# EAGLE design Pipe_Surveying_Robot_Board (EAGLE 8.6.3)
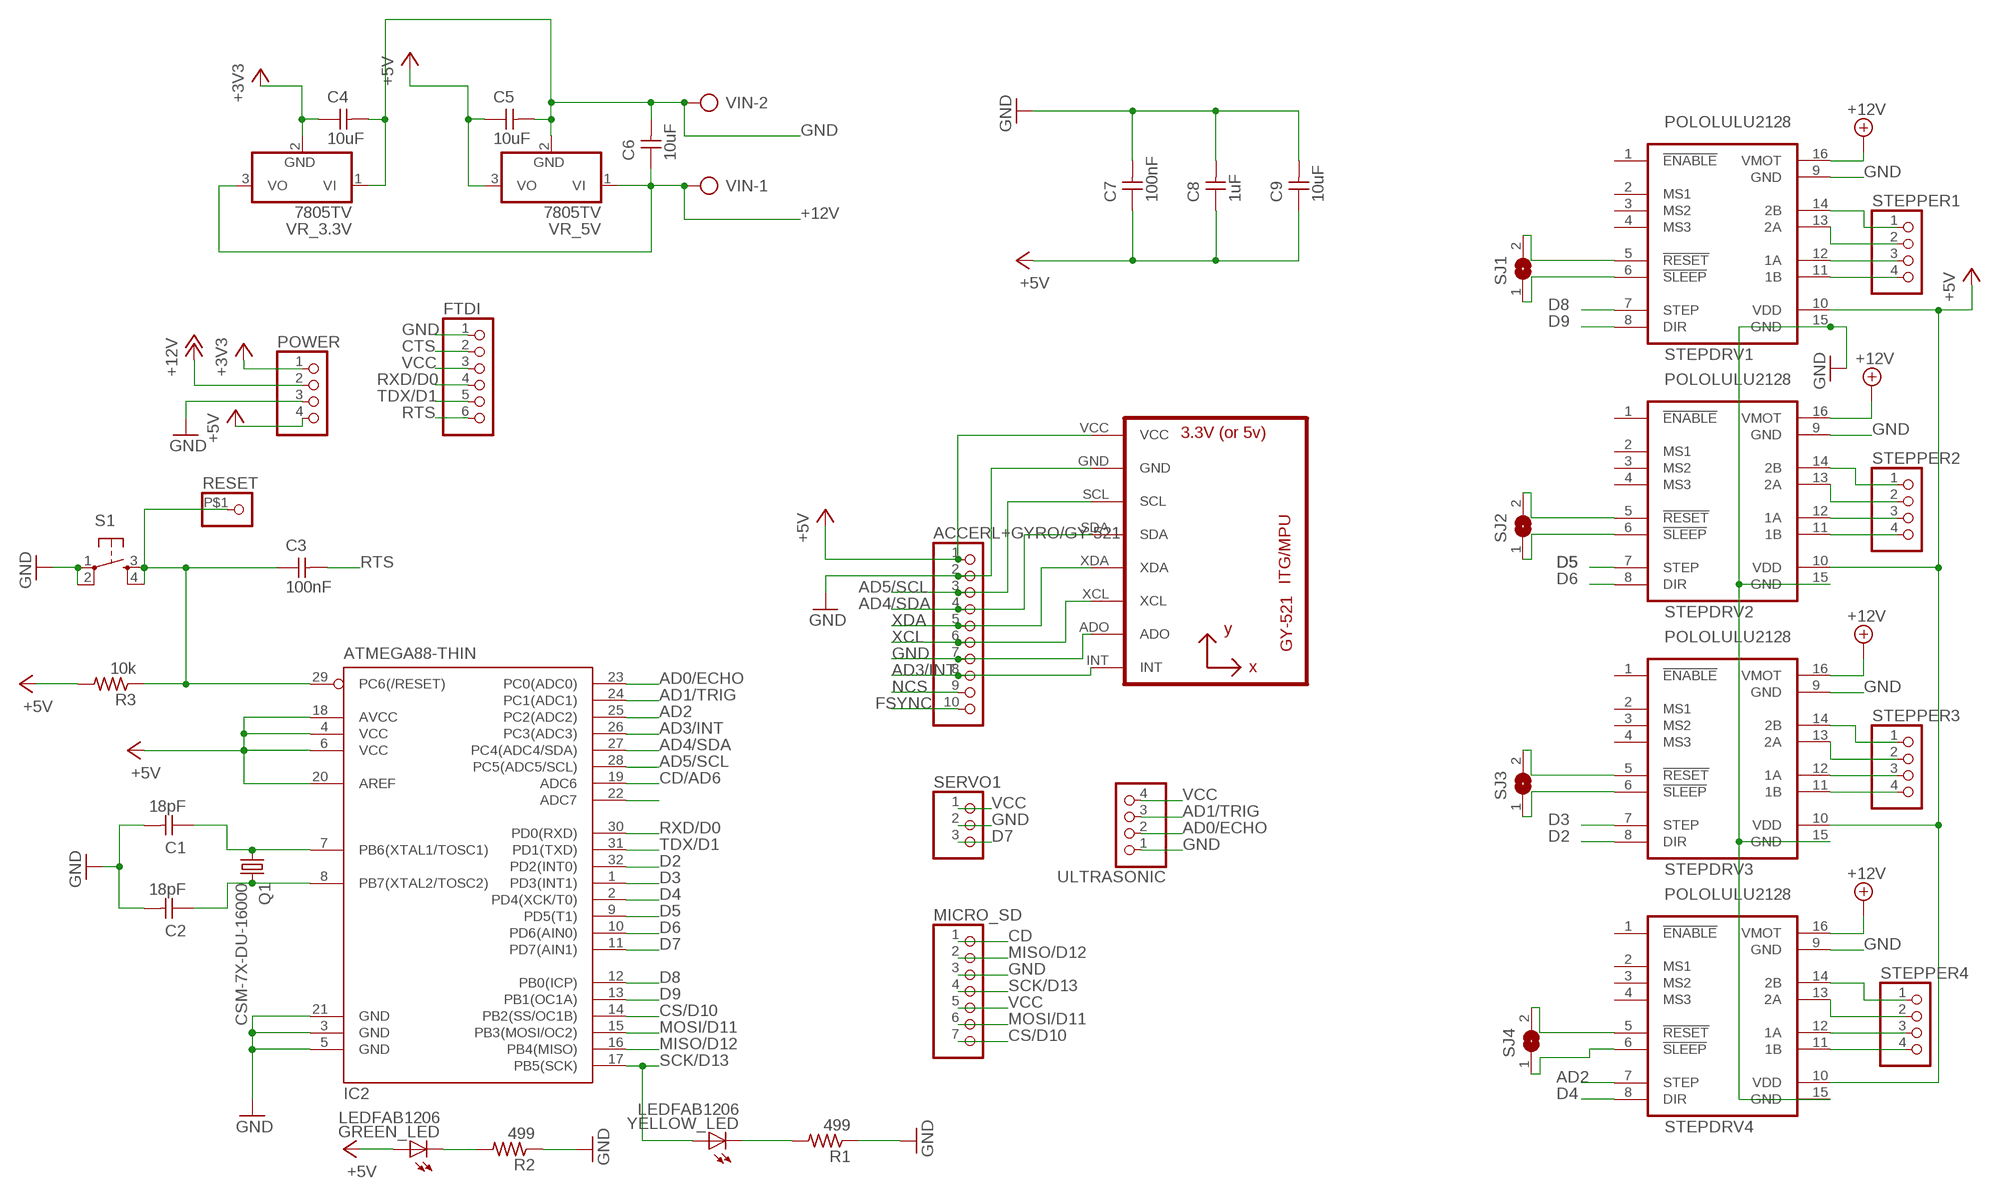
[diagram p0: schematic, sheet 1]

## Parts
ACCERL+GYRO/GY-521  PINHD-1X10  [1X10]
C1  18pF  CAP-UNPOLARIZED  [C1206]
C2  18pF  CAP-UNPOLARIZED  [C1206]
C3  100nF  CAP-UNPOLARIZEDFAB  [C1206FAB]
C4  10uF  CAP-UNPOLARIZEDFAB  [C1206FAB]
C5  10uF  CAP-UNPOLARIZEDFAB  [C1206FAB]
C6  10uF  CAP-UNPOLARIZEDFAB  [C1206FAB]
C7  100nF  CAP-UNPOLARIZEDFAB  [C1206FAB]
C8  1uF  CAP-UNPOLARIZEDFAB  [C1206FAB]
C9  10uF  CAP-UNPOLARIZEDFAB  [C1206FAB]
FTDI  PINHD-1X6  [1X06]
GREEN_LED  LEDFAB1206  [LED1206FAB]
IC2  ATMEGA88-THIN  [TQFP32-08THIN]
MICRO_SD  PINHD-1X7  [1X07]
POWER  PINHD-1X4  [1X04]
Q1  CSM-7X-DU-16000  CSM-7X-DU  [CSM-7X-DU]
R1  499  RES-US1206FAB  [R1206FAB]
R2  499  RES-US1206FAB  [R1206FAB]
R3  10k  RES-US1206FAB  [R1206FAB]
RESET  PINHD-1X1-BIGPOGO  [1X1-BIGPOGO]
S1  6MM_SWITCH6MM_SWITCH  [6MM_SWITCH]
SERVO1  PINHD-1X3  [1X03]
SJ1  SJ  [SJ]
SJ2  SJ  [SJ]
SJ3  SJ  [SJ]
SJ4  SJ  [SJ]
STEPDRV1  POLOLULU2128  [POLOLULU2128]
STEPDRV2  POLOLULU2128  [POLOLULU2128]
STEPDRV3  POLOLULU2128  [POLOLULU2128]
STEPDRV4  POLOLULU2128  [POLOLULU2128]
STEPPER1  PINHD-1X4  [1X04]
STEPPER2  PINHD-1X4  [1X04]
STEPPER3  PINHD-1X4  [1X04]
STEPPER4  PINHD-1X4  [1X04]
U1  GY-521MPU6050  [GY-521]
ULTRASONIC  PINHD-1X4  [1X04]
VIN  AK500/2  [AK500/2]
VR_3.3V  7805TV  [TO220V]
VR_5V  7805TV  [TO220V]
YELLOW_LED  LEDFAB1206  [LED1206FAB]

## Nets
+3V3: C4.1 POWER.1 VR_3.3V.2(GND)
+12V: C6.1 POWER.2 STEPDRV1.16(VMOT) STEPDRV2.16(VMOT) STEPDRV3.16(VMOT) STEPDRV4.16(VMOT) VIN.1 VR_3.3V.3(VO) VR_5V.1(VI)
AD0/ECHO: IC2.23(PC0(ADC0)) ULTRASONIC.2
AD1/TRIG: IC2.24(PC1(ADC1)) ULTRASONIC.3
AD2: IC2.25(PC2(ADC2)) STEPDRV4.7(STEP)
AD3/INT: ACCERL+GYRO/GY-521.8 IC2.26(PC3(ADC3)) U1.INT
AD4/SDA: ACCERL+GYRO/GY-521.4 IC2.27(PC4(ADC4/SDA)) U1.SDA
AD5/SCL: ACCERL+GYRO/GY-521.3 IC2.28(PC5(ADC5/SCL)) U1.SCL
AD7/TRIG: IC2.22(ADC7)
CD: MICRO_SD.1
CD/AD6: IC2.19(ADC6)
CS/D10: IC2.14(PB2(SS/OC1B)) MICRO_SD.7
CTS: FTDI.2
D2: IC2.32(PD2(INT0)) STEPDRV3.8(DIR)
D3: IC2.1(PD3(INT1)) STEPDRV3.7(STEP)
D4: IC2.2(PD4(XCK/T0)) STEPDRV4.8(DIR)
D5: IC2.9(PD5(T1)) STEPDRV2.7(STEP)
D6: IC2.10(PD6(AIN0)) STEPDRV2.8(DIR)
D7: IC2.11(PD7(AIN1)) SERVO1.3
D8: IC2.12(PB0(ICP)) STEPDRV1.7(STEP)
D9: IC2.13(PB1(OC1A)) STEPDRV1.8(DIR)
FSYNC: ACCERL+GYRO/GY-521.10
GND: ACCERL+GYRO/GY-521.2 ACCERL+GYRO/GY-521.7 C1.2 C2.2 C4.2 C5.2 C6.2 C7.2 C8.2 C9.2 FTDI.1 IC2.3(GND) IC2.5(GND) IC2.21(GND) MICRO_SD.3 POWER.3 R1.1 R2.1 S1.1(P) S1.2(P1) SERVO1.2 STEPDRV1.9(GND) STEPDRV1.15(GND) STEPDRV2.9(GND) STEPDRV2.15(GND) STEPDRV3.9(GND) STEPDRV3.15(GND) STEPDRV4.9(GND) STEPDRV4.15(GND) U1.ADO U1.GND ULTRASONIC.1 VIN.2 VR_3.3V.1(VI) VR_5V.2(GND)
MISO/D12: IC2.16(PB4(MISO)) MICRO_SD.2
MOSI/D11: IC2.15(PB3(MOSI/OC2)) MICRO_SD.6
N$1: STEPDRV1.11(1B) STEPPER1.4
N$2: STEPDRV1.12(1A) STEPPER1.3
N$3: R1.2 YELLOW_LED.2(C)
N$4: STEPDRV1.13(2A) STEPPER1.2
N$5: C2.1 IC2.8(PB7(XTAL2/TOSC2)) Q1.2
N$6: C1.1 IC2.7(PB6(XTAL1/TOSC1)) Q1.1
N$7: STEPDRV1.14(2B) STEPPER1.1
N$8: STEPDRV4.11(1B) STEPPER4.4
N$9: STEPDRV4.12(1A) STEPPER4.3
N$10: STEPDRV4.13(2A) STEPPER4.2
N$11: STEPDRV4.14(2B) STEPPER4.1
N$12: STEPDRV3.11(1B) STEPPER3.4
N$13: STEPDRV3.12(1A) STEPPER3.3
N$14: STEPDRV3.13(2A) STEPPER3.2
N$15: STEPDRV3.14(2B) STEPPER3.1
N$16: STEPDRV2.11(1B) STEPPER2.4
N$17: STEPDRV2.12(1A) STEPPER2.3
N$18: STEPDRV2.13(2A) STEPPER2.2
N$19: STEPDRV2.14(2B) STEPPER2.1
N$20: SJ1.1 STEPDRV1.6(!SLEEP)
N$21: SJ1.2 STEPDRV1.5(!RESET)
N$22: SJ4.1 STEPDRV4.6(!SLEEP)
N$23: SJ4.2 STEPDRV4.5(!RESET)
N$24: SJ3.2 STEPDRV3.5(!RESET)
N$25: SJ3.1 STEPDRV3.6(!SLEEP)
N$26: SJ2.2 STEPDRV2.5(!RESET)
N$27: SJ2.1 STEPDRV2.6(!SLEEP)
N$34: GREEN_LED.2(C) R2.2
NCS: ACCERL+GYRO/GY-521.9
RESET: C3.1 IC2.29(PC6(/RESET)) R3.1 RESET.P$1 S1.3(S) S1.4(S1)
RTS: C3.2 FTDI.6
RXD/D0: FTDI.4 IC2.30(PD0(RXD))
SCK/D13: IC2.17(PB5(SCK)) MICRO_SD.4 YELLOW_LED.1(A)
TDX/D1: FTDI.5 IC2.31(PD1(TXD))
VCC: ACCERL+GYRO/GY-521.1 C5.1 C7.1 C8.1 C9.1 FTDI.3 GREEN_LED.1(A) IC2.4(VCC) IC2.6(VCC) IC2.18(AVCC) IC2.20(AREF) MICRO_SD.5 POWER.4 R3.2 SERVO1.1 STEPDRV1.10(VDD) STEPDRV2.10(VDD) STEPDRV3.10(VDD) STEPDRV4.10(VDD) U1.VCC ULTRASONIC.4 VR_5V.3(VO) ; supply symbol labelled +5V
XCL: ACCERL+GYRO/GY-521.6 U1.XCL
XDA: ACCERL+GYRO/GY-521.5 U1.XDA
Unconnected: STEPDRV1.1(!ENABLE) STEPDRV1.2(MS1) STEPDRV1.3(MS2) STEPDRV1.4(MS3) STEPDRV2.1(!ENABLE) STEPDRV2.2(MS1) STEPDRV2.3(MS2) STEPDRV2.4(MS3) STEPDRV3.1(!ENABLE) STEPDRV3.2(MS1) STEPDRV3.3(MS2) STEPDRV3.4(MS3) STEPDRV4.1(!ENABLE) STEPDRV4.2(MS1) STEPDRV4.3(MS2) STEPDRV4.4(MS3)

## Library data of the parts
ACCERL+GYRO/GY-521 = pinhead:PINHD-1X10: PIN HEADER
C1-C9 = fab:CAP-UNPOLARIZED
FTDI = pinhead:PINHD-1X6: PIN HEADER
GREEN_LED YELLOW_LED = fab:LED: LED
IC2 = fab:ATMEGA88-THIN
MICRO_SD = pinhead:PINHD-1X7: PIN HEADER
POWER STEPPER1-STEPPER4 ULTRASONIC = pinhead:PINHD-1X4: PIN HEADER
Q1 = crystal:CSM-7X-DU: SMD CRYSTAL; OC_FARNELL: unknown; OC_NEWARK: unknown
R1-R3 = fab:RES-US: Resistor (US Symbol)
RESET = adafruit:PINHD-1X1: Pin header 1x1 for 0.1" spacing
S1 = fab:6MM_SWITCH: OMRON SWITCH
SERVO1 = pinhead:PINHD-1X3: PIN HEADER
SJ1-SJ4 = jumper:SJ: SMD solder JUMPER
STEPDRV1-STEPDRV4 = stepper_drivers_etc:POLOLULU2128
U1 = gy-521:GY-521
VIN = con-ptr500:AK500/2: CONNECTOR; OC_FARNELL: unknown; OC_NEWARK: unknown
VR_3.3V VR_5V = linear:78*: Positive VOLTAGE REGULATOR Source: http://cache.national.com/ds/LM/LM78L05.pdf http://www.fairchildsemi.com/ds/LM/LM7805.pdf

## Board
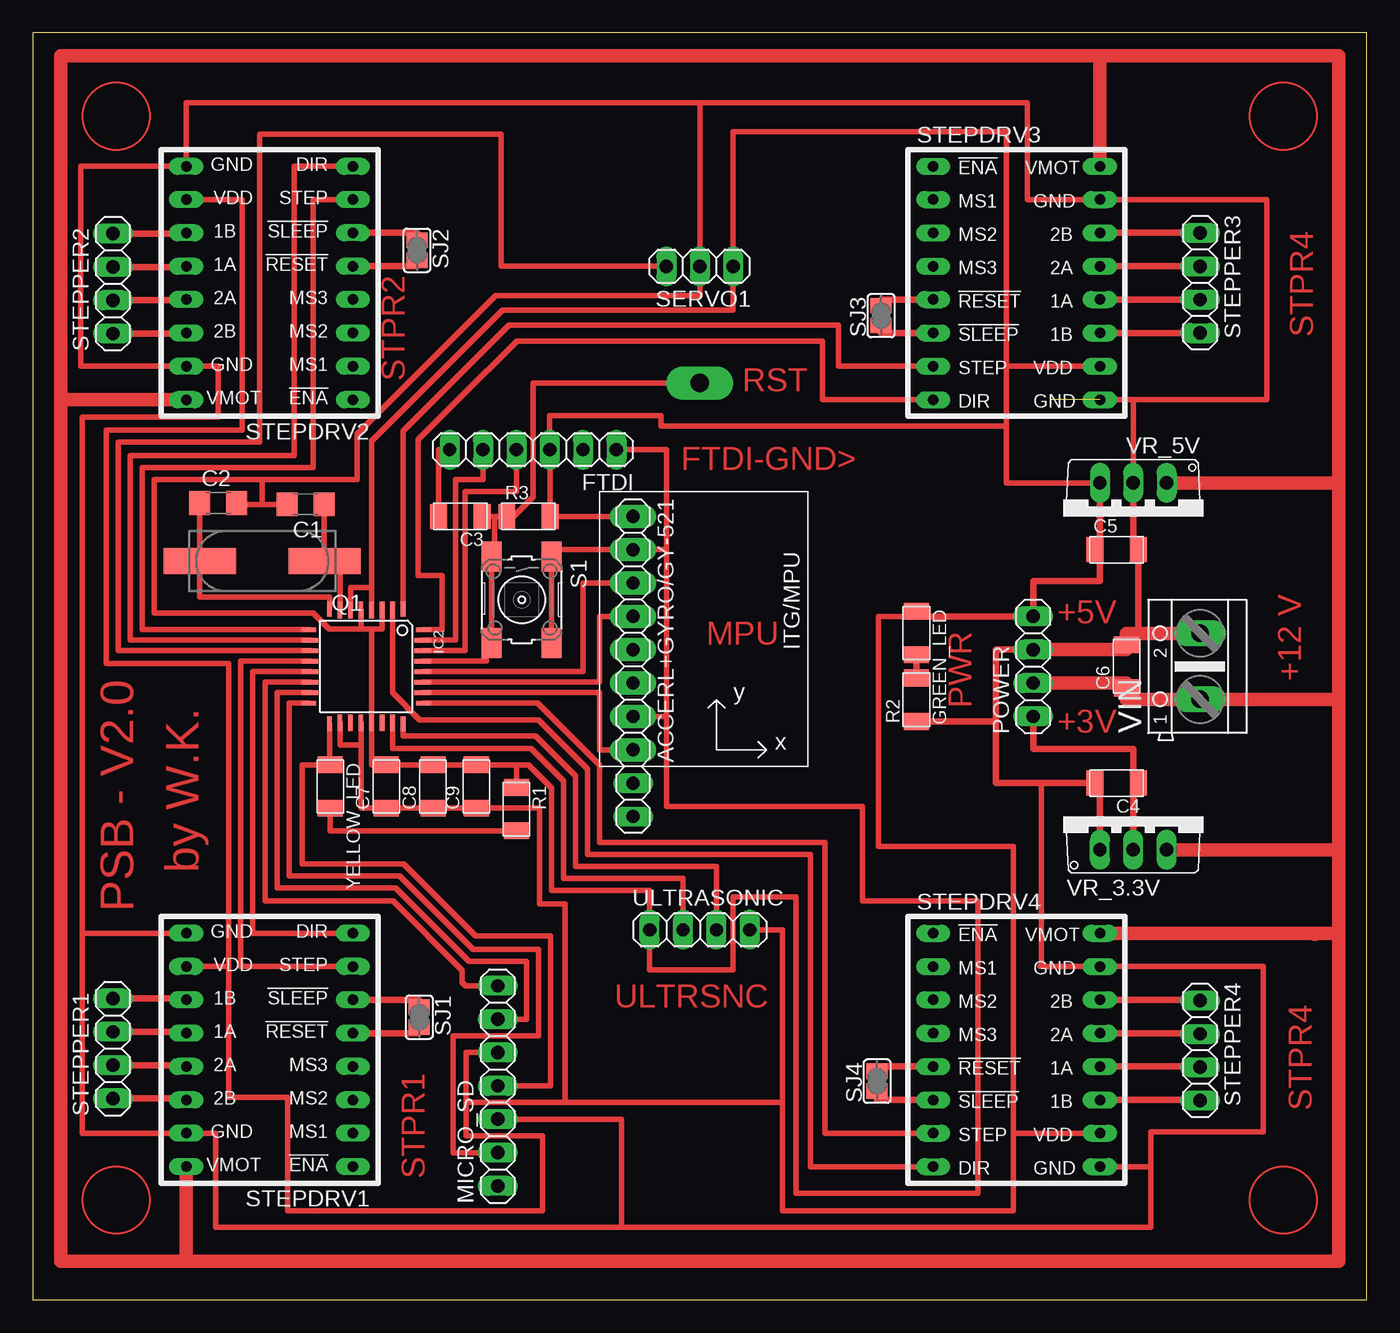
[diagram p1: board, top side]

Size 101.6 x 96.52 mm. Coordinates in mm from the lower left corner, seen from the top.
Outline: 0,0 101.6,0 101.6,96.52 0,96.52 0,0
Copper layers (1*16): Top 0.035mm / dielectric 1.5mm / Bottom 0.035mm
Design rules "default": minimum track width 6mil, minimum drill 0.35mm, track to track 6mil, track to pad 6mil, pad to pad 6mil, via to via 6mil, smd to smd 6mil, copper to edge 40mil, drill to drill 6mil, minimum pad ring 10mil, minimum via ring 8mil, stop-mask expansion 4mil, vias tented up to drill 0mil, thermal gap 10mil

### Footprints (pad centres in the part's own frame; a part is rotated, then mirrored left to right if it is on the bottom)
1X10 = drill 1.016 long: 1 -11.43,0; 2 -8.89,0; 3 -6.35,0; 4 -3.81,0; 5 -1.27,0; 6 1.27,0; 7 3.81,0; 8 6.35,0; 9 8.89,0; 10 11.43,0
C1206 = smd 1.6 x 1.8: 1 -1.4,0; 2 1.4,0
C1206FAB = smd 1.27 x 1.905: 1 -1.651,0; 2 1.651,0
1X06 = drill 1.016 long: 1 -6.35,0; 2 -3.81,0; 3 -1.27,0; 4 1.27,0; 5 3.81,0; 6 6.35,0
LED1206FAB = smd 1.27 x 1.905: 1 -1.651,0; 2 1.651,0
TQFP32-08THIN = smd 1.118 x 0.356: 1 -4.369,2.8; 8 -4.369,-2.8; 17 4.369,-2.8; 24 4.369,2.8 | smd 1.27 x 0.356: 2 -4.293,2; 3 -4.293,1.2; 4 -4.293,0.4; 5 -4.293,-0.4; 6 -4.293,-1.2; 7 -4.293,-2; 18 4.293,-2; 19 4.293,-1.2; 20 4.293,-0.4; 21 4.293,0.4; 22 4.293,1.2; 23 4.293,2 | smd 0.356 x 1.118: 9 -2.8,-4.369; 16 2.8,-4.369; 25 2.8,4.369; 32 -2.8,4.369 | smd 0.356 x 1.27: 10 -2,-4.293; 14 1.2,-4.293; 15 2,-4.293; 26 2,4.293; 27 1.2,4.293; 31 -2,4.293 | smd 0.35 x 1.27: 11 -1.2,-4.293; 12 -0.4,-4.293; 13 0.4,-4.293; 28 0.4,4.293; 29 -0.4,4.293; 30 -1.2,4.293
1X07 = drill 1.016 long: 1 -7.62,0; 2 -5.08,0; 3 -2.54,0; 4 0,0; 5 2.54,0; 6 5.08,0; 7 7.62,0
1X04 = drill 1.016 long: 1 -3.81,0; 2 -1.27,0; 3 1.27,0; 4 3.81,0
CSM-7X-DU = smd 5.5 x 2: 1 -4.75,0; 2 4.75,0
R1206FAB = smd 1.27 x 1.905: 1 -1.651,0; 2 1.651,0
1X1-BIGPOGO = drill 1.4 pad 2.54 long: P$1 0,0
6MM_SWITCH = smd 2.286 x 1.524: 1 -3.302,2.286; 2 3.302,2.286; 3 -3.302,-2.286; 4 3.302,-2.286
1X03 = drill 1.016 long: 1 -2.54,0; 2 0,0; 3 2.54,0
SJ = smd 1.168 x 1.6: 1 -0.762,0; 2 0.762,0
POLOLULU2128 = drill 0.8 long: 1 -7.62,7.62; 2 -7.62,5.08; 3 -7.62,2.54; 4 -7.62,0; 5 -7.62,-2.54; 6 -7.62,-5.08; 7 -7.62,-7.62; 8 -7.62,-10.16; 9 5.08,-10.16; 10 5.08,-7.62; 11 5.08,-5.08; 12 5.08,-2.54; 13 5.08,0; 14 5.08,2.54; 15 5.08,5.08; 16 5.08,7.62
GY-521 = drill 0.8 pad 1.778 long: ADO -8.89,-6.35; GND -8.89,6.35; INT -8.89,-8.89; SCL -8.89,3.81; SDA -8.89,1.27; VCC -8.89,8.89; XCL -8.89,-3.81; XDA -8.89,-1.27
AK500/2 = drill 1.321 long: 1 -2.515,0; 2 2.515,0
TO220V = drill 1.016 long: 1 -2.54,-2.54; 2 0,-2.54; 3 2.54,-2.54

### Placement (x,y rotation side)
ACCERL+GYRO/GY-521  45.72,48.26 270 top
C1  20.78,60.6 180 top
C2  14.12,60.71 0 top
C3  32.56,59.69 180 top
C4  82.55,39.37 180 top
C5  82.55,57.15 0 top
C6  83.31,48.26 90 top
C7  26.92,39.12 90 top
C8  30.48,39.12 90 top
C9  33.78,39.12 90 top
FTDI  38.1,64.77 180 top
GREEN_LED  67.31,50.8 270 top
IC2  25.4,48.26 270 top
MICRO_SD  35.41,16.31 90 top
POWER  76.2,48.26 90 top
Q1  17.48,56.29 180 top
R1  36.83,37.39 270 top
R2  67.31,45.72 90 top
R3  37.74,59.69 0 top
RESET  50.8,69.85 0 top
S1  37.24,53.34 270 top
SERVO1  50.8,78.74 180 top
SJ1  29.44,21.54 270 top
SJ2  29.26,79.96 270 top
SJ3  64.62,74.98 90 top
SJ4  64.31,16.66 90 top
STEPDRV1  16.76,17.78 180 top
STEPDRV2  16.76,76.2 180 top
STEPDRV3  76.2,78.74 0 top
STEPDRV4  76.2,20.32 0 top
STEPPER1  6.1,19.15 90 top
STEPPER2  6.1,77.42 90 top
STEPPER3  88.9,77.47 270 top
STEPPER4  88.9,19 270 top
U1  54.61,50.8 0 top
ULTRASONIC  50.8,28.19 0 top
VIN  88.9,48.26 90 top
VR_3.3V  83.82,36.83 0 top
VR_5V  83.82,59.69 180 top
YELLOW_LED  22.66,39.12 270 top

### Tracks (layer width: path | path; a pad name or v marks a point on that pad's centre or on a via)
+3V3
  Top 0.508: VR_3.3V.2 83.82,38.1 83.82,39.37 | 83.82,39.37 C4.1 | 83.82,39.37 83.82,41.96 76.2,41.96 POWER.1
+12V
  Top 1.016: 99.47,45.74 VIN.1 83.31,45.74 C6.1 83.31,46.99 POWER.2 | 11.68,2.95 2.13,2.95 2.13,68.58 | STEPDRV2.16 2.13,68.58 | STEPDRV1.16 11.68,2.95 | 2.13,68.58 2.13,94.79 81.28,94.79 | VR_5V.1 99.47,62.23 | VR_3.3V.3 99.47,34.29 | STEPDRV4.16 96.62,27.94 97.64,27.94 | 97.64,27.94 97.64,27.84 | 81.28,94.79 99.47,94.79 99.47,62.23 | 11.68,2.95 99.47,2.95 99.47,27.94 | 99.47,27.94 99.47,34.29 | 99.47,34.29 99.47,45.74 | 99.47,45.74 99.47,62.23 | STEPDRV3.16 81.28,94.79 | 97.64,27.94 99.47,27.94
AD0/ECHO
  Top 0.406: IC2.23 27.4,42.16 27.4,42.01 37.95,42.01 40.44,39.52 40.44,32.11 49.53,32.11 ULTRASONIC.2
AD1/TRIG
  Top 0.406: IC2.24 28.2,42.98 38.3,42.98 41.35,39.93 41.35,33.02 52.07,33.02 ULTRASONIC.3
AD2
  Top 0.406: STEPDRV4.7 63.4,12.7 62.08,12.7 60.35,12.7 60.35,34.85 43.18,34.85 43.18,40.74 38.46,45.46 IC2.25
AD3/INT
  Top 0.406: IC2.26 43.18,46.26 43.18,41.91 U1.INT
AD4/SDA
  Top 0.406: U1.SDA 43.18,52.07 43.18,47.06 IC2.27
AD5/SCL
  Top 0.406: IC2.28 41.91,47.86 41.91,54.61 U1.SCL
CS/D10
  Top 0.406: MICRO_SD.7 32.97,23.93 32.72,24.18 32.72,25.1 27.43,30.38 17.68,30.38 17.68,47.06 IC2.14
D2
  Top 0.406: IC2.32 31.19,51.06 31.19,55.17 29.36,55.17 29.36,65.53 32.05,68.22 32.41,68.58 36.88,73.05 60.15,73.05 60.15,68.58 STEPDRV3.8
D3
  Top 0.406: IC2.1 28.2,66.2 36.27,74.27 51.51,74.27 61.37,74.27 61.37,71.12 STEPDRV3.7
D4
  Top 0.406: IC2.2 27.4,46.26 29.46,44.2 38.51,44.2 42.27,40.44 42.27,33.93 59.23,33.93 59.23,10.16 59.44,10.16 60.86,10.16 STEPDRV4.8
D5
  Top 0.406: STEPDRV2.7 21.34,83.82 21.34,65.23 21.34,64.52 21.34,63.4 8.33,63.4 8.33,51.06 IC2.9
D6
  Top 0.406: STEPDRV2.8 19.91,86.36 19.91,65.63 19.91,65.43 19.91,64.31 7.42,64.31 7.42,50.26 IC2.10
D7
  Top 0.406: IC2.11 6.5,49.46 6.5,65.33 17.27,65.33 17.27,88.8 35.66,88.8 35.66,78.74 SERVO1.3
D8
  Top 0.406: IC2.12 15.85,48.66 15.85,25.4 STEPDRV1.7
D9
  Top 0.406: IC2.13 16.76,47.86 16.76,27.94 STEPDRV1.8
GND  (1 unrouted)
  Top 0.406: 48.26,57.15 U1.GND 39.52,57.15 S1.1 S1.2 | 48.26,57.15 48.26,44.45 | 48.26,44.45 U1.ADO | FTDI.1 48.26,64.77 48.26,57.15 | C2.2 15.52,60.6 17.48,60.6 | 17.48,60.6 C1.2 | 36.83,40.77 C9.2 C8.2 C7.2 25.8,40.77 IC2.21 25.8,49.89 25.8,51.11 | R1.1 36.83,40.77 | 76.81,25.4 STEPDRV4.15 93.73,25.4 93.73,12.8 85.14,12.8 85.14,10.16 | 76.81,25.4 76.71,25.4 | 83.82,68.58 93.98,68.58 93.98,83.82 STEPDRV3.15 75.74,83.82 75.74,91.19 50.8,91.19 | 83.82,68.58 STEPDRV3.9 | 50.8,91.19 SERVO1.2 50.8,76.5 35.26,76.5 24.69,65.94 24.69,62.48 17.48,62.48 | 50.8,91.19 11.68,91.19 STEPDRV2.9 3.66,86.36 3.66,71.12 STEPDRV2.15 14.12,71.12 14.12,67.26 3.76,67.26 3.76,27.94 | MICRO_SD.3 44.86,13.77 44.86,5.54 | 44.86,5.54 13.92,5.54 13.92,12.7 STEPDRV1.15 3.76,12.7 3.76,27.94 | 36.83,40.77 37.77,40.77 39.52,39.01 39.52,31.19 46.99,31.19 ULTRASONIC.1 46.99,25.15 53.34,25.15 53.34,30.68 58.12,30.68 58.12,8.13 71.98,8.13 71.98,30.38 63.2,30.38 63.2,37.59 48.26,37.59 48.26,44.45 | 3.76,27.94 STEPDRV1.9 | 17.48,60.6 17.48,62.48 | 25,51.11 22.55,51.11 21.34,52.32 9.25,52.32 9.25,62.48 17.48,62.48 | 25,51.11 25.8,51.11 | 25.8,51.11 26.6,51.11 IC2.3 | IC2.5 25,51.11 | 76.81,25.4 76.81,39.37 76.71,39.37 | VR_5V.2 83.82,68.58 | STEPDRV4.9 85.14,10.16 | 85.14,10.16 85.14,5.54 44.86,5.54
  Top 0.508: VR_3.3V.1 81.28,39.37 C4.2 76.71,39.37 73.36,39.37 73.36,44.07 | VR_5V.2 83.82,57.15 C5.2 84.2,50.77 84.23,50.77 | POWER.3 73.36,49.53 73.36,44.07 | R2.1 73.36,44.07
  Top 1.016: VIN.2 84.23,50.77 83.31,50.77 C6.2 83.31,49.53 POWER.3
MISO/D12
  Top 0.406: MICRO_SD.2 32,11.23 32,20.12 38.51,20.12 38.51,26.72 33.53,26.72 27.94,32.31 19.51,32.31 19.51,42.67 19.51,42.88 19.51,45.46 IC2.16
MOSI/D11
  Top 0.406: MICRO_SD.6 37.59,21.39 37.59,25.81 33.22,25.81 28.14,30.89 27.84,31.19 27.64,31.39 18.59,31.39 18.59,46.26 IC2.15
N$1
  Top 0.508: STEPPER1.4 12.7,22.96 STEPDRV1.11
N$2
  Top 0.508: STEPPER1.3 12.7,20.42 STEPDRV1.12
N$3
  Top 0.406: R1.2 22.66,35.74 YELLOW_LED.2
N$4
  Top 0.508: STEPPER1.2 12.7,17.88 STEPDRV1.13
N$5
  Top 0.406: C2.1 Q1.2 12.72,53.54 22.6,53.54 IC2.8
N$6
  Top 0.406: C1.1 22.18,56.29 Q1.1 23.4,56.29 | 24.01,56.29 23.47,56.29 23.4,56.29 | IC2.7 23.4,56.29
N$7
  Top 0.508: STEPPER1.1 12.7,15.34 STEPDRV1.14
N$8
  Top 0.508: STEPDRV4.11 88.9,15.24 STEPPER4.4
N$9
  Top 0.508: STEPDRV4.12 88.9,17.78 STEPPER4.3
N$10
  Top 0.508: STEPDRV4.13 88.9,20.32 STEPPER4.2
N$11
  Top 0.508: STEPDRV4.14 88.9,22.86 STEPPER4.1
N$12
  Top 0.508: STEPDRV3.11 STEPPER3.4
N$13
  Top 0.508: STEPDRV3.12 STEPPER3.3
N$14
  Top 0.508: STEPDRV3.13 STEPPER3.2
N$15
  Top 0.508: STEPDRV3.14 STEPPER3.1
N$16
  Top 0.508: STEPPER2.4 12.7,81.23 STEPDRV2.11
N$17
  Top 0.508: STEPDRV2.12 12.7,78.69 STEPPER2.3
N$18
  Top 0.508: STEPPER2.2 12.7,76.15 STEPDRV2.13
N$19
  Top 0.508: STEPPER2.1 12.7,73.61 STEPDRV2.14
N$20
  Top 0.508: STEPDRV1.6 29.44,22.86 SJ1.1
N$21
  Top 0.508: STEPDRV1.5 29.44,20.32 SJ1.2
N$22
  Top 0.508: STEPDRV4.6 64.31,15.24 SJ4.1
N$23
  Top 0.508: STEPDRV4.5 64.31,17.78 SJ4.2
N$24
  Top 0.508: STEPDRV3.5 64.62,76.2 SJ3.2
N$25
  Top 0.508: STEPDRV3.6 64.62,73.66 SJ3.1
N$26
  Top 0.508: STEPDRV2.5 29.26,78.74 SJ2.2
N$27
  Top 0.508: STEPDRV2.6 29.26,81.28 SJ2.1
N$34
  Top 0.508: GREEN_LED.2 R2.2
RESET
  Top 0.406: IC2.29 34.54,48.66 34.54,49.78 S1.4 S1.3 35.15,56.64 35.15,59.69 | C3.1 35.15,59.69 | 35.15,59.69 R3.1 36.63,59.69 38.1,61.16 38.1,69.85 RESET.P$1
RTS
  Top 0.406: 30.89,59.69 C3.2 30.91,64.77 FTDI.6
RXD/D0
  Top 0.406: FTDI.4 36.83,61.57 32.92,61.57 32.92,49.46 IC2.30
SCK/D13
  Top 0.406: IC2.17 22.6,41.58 YELLOW_LED.1 20.52,40.77 20.52,33.22 28.25,33.22 33.73,27.74 39.42,27.74 39.42,16.31 MICRO_SD.4
TDX/D1
  Top 0.406: FTDI.5 34.29,62.48 32.21,62.48 32.21,50.26 IC2.31
VCC
  Top 0.406: U1.VCC R3.2 39.4,64.77 FTDI.3 39.37,67.36 47.85,67.36 47.85,66.55 74.17,66.55 | IC2.20 25,42.27 | 25,42.27 25,41.45 25,37.47 C7.1 C8.1 C9.1 38.61,37.47 38.61,30.18 40.54,30.18 40.54,15.04 | 74.68,12.7 STEPDRV4.10 | 74.68,12.7 74.68,6.81 57.1,6.81 57.1,15.04 | MICRO_SD.5 33.02,18.85 33.02,15.04 | 33.02,15.04 40.54,15.04 | IC2.18 23.4,42.27 25,42.27 | STEPDRV2.10 15.95,83.82 15.95,66.24 5.59,66.24 5.59,48.46 14.94,48.46 14.94,25.4 | 14.94,25.4 STEPDRV1.10 | 14.94,25.4 14.94,15.44 19.41,15.44 19.41,6.81 38.81,6.81 38.81,12.5 33.02,12.5 33.02,15.04 | IC2.6 24.2,54.25 25.8,54.25 | 25.8,54.25 25.8,53.85 IC2.4 | 74.17,71.12 STEPDRV3.10 | 74.17,66.55 74.17,71.12 | 74.17,71.12 74.17,89 53.34,89 SERVO1.1 53.34,75.39 35.76,75.39 25.8,65.42 25.8,54.25 | 74.68,12.7 74.68,34.54 64.41,34.54 64.41,52.07 67.31,52.07 | VR_5V.3 74.17,62.23 74.17,66.55 | 40.54,15.04 57.1,15.04 | ULTRASONIC.4 57.1,28.19 57.1,15.04
  Top 0.508: VR_5V.3 81.28,57.15 | C5.1 81.28,57.15 | 81.28,57.15 81.28,54.76 76.2,54.76 POWER.4 67.31,52.07 GREEN_LED.1
(copper drawn outside any net)
  shapes: Top circle x4

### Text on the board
Top: STPR4 | STPR2 | RST | FTDI-GND> | +5V | MPU | +12 V | PWR | +3V | by W.K. | PSB - V2.0 | ULTRSNC | STPR4 | STPR1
